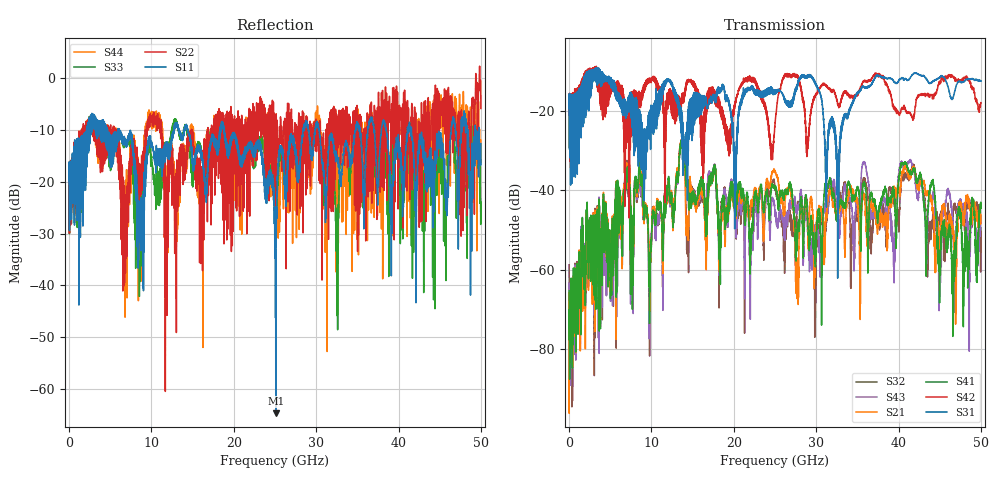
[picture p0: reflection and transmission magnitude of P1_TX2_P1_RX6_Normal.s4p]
!Keysight Technologies,N5225B,MY57041031,A.13.20.10
!Date: Friday, May 31, 2019 11:22:18
!Correction: S11(Full 4 Port(1,2,3,4))
!S12(Full 4 Port(1,2,3,4))
!S13(Full 4 Port(1,2,3,4))
!S14(Full 4 Port(1,2,3,4))
!S21(Full 4 Port(1,2,3,4))
!S22(Full 4 Port(1,2,3,4))
!S23(Full 4 Port(1,2,3,4))
!S24(Full 4 Port(1,2,3,4))
!S31(Full 4 Port(1,2,3,4))
!S32(Full 4 Port(1,2,3,4))
!S33(Full 4 Port(1,2,3,4))
!S34(Full 4 Port(1,2,3,4))
!S41(Full 4 Port(1,2,3,4))
!S42(Full 4 Port(1,2,3,4))
!S43(Full 4 Port(1,2,3,4))
!S44(Full 4 Port(1,2,3,4))
!S4P File: Measurements: <S11,S12,S13,S14>,
!<S21,S22,S23,S24>,
!<S31,S32,S33,S34>,
!<S41,S42,S43,S44>:
# Hz S  dB  R 50.0
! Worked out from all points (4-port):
!   5000 points, 10 MHz to 50 GHz, reference 50 ohm
!   strongest paths, dB at 10 MHz, 12.51 GHz, 25.01 GHz, 37.51 GHz, 50 GHz:
!     S31: -19.4, -13.0, -15.4, -11.1, -12.5
!     S42: -19.4, -15.7, -23.1, -11.0, -18.0
!     S41: -65.3, -43.8, -39.4, -46.0, -44.0
!     S21: -68.2, -43.4, -35.5, -48.1, -46.1
!     S43: -63.4, -43.6, -44.9, -45.8, -48.2
!     S32: -58.7, -43.2, -38.8, -45.6, -55.4
!   lowest |S11| = -64.6 dB at 25.1 GHz (marker M1), VSWR 1.00, Z = 49.9 + j0.0148 ohm
!   |S11| at or under -10 dB: 6.091 GHz to 12.71 GHz (6.616 GHz wide, 70.4 % of centre); 18.82 GHz to 28.43 GHz (9.604 GHz wide, 40.7 % of centre); 41.58 GHz to 46.39 GHz (4.811 GHz wide, 10.9 % of centre)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
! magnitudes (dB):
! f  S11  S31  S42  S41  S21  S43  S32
! 10 MHz  -19.8  -19.4  -19.4  -65.3  -68.2  -63.4  -58.7
! 13.72 GHz  -11.8  -29.0  -17.1  -27.1  -27.4  -27.6  -27.5
! 14.39 GHz  -9.8  -27.6  -12.2  -37.9  -48.4  -37.9  -49.9
! 25.1 GHz  -64.6  -15.1  -21.3  -39.5  -35.7  -46.2  -39.8
! 27.66 GHz  -16.1  -14.2  -11.3  -53.2  -61.2  -44.3  -45.4
! 32.64 GHz  -15.8  -37.6  -18.4  -45.9  -46.0  -45.5  -45.2
! 50 GHz  -12.7  -12.5  -18.0  -44.0  -46.1  -48.2  -55.4
